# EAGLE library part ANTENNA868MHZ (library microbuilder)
868MHz Surface-Mount Antenna Digikey: ANT-868-SP_-ND
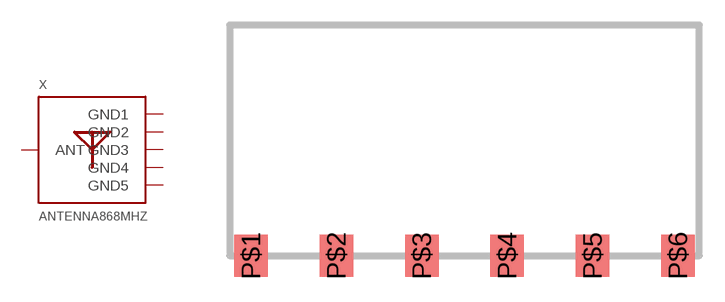
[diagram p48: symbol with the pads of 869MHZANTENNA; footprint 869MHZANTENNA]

Designator prefix X

## ANTENNA868MHZ  [869MHZANTENNA]
P$1  ANT
P$2  GND1  pwr
P$3  GND2  pwr
P$4  GND3  pwr
P$5  GND4  pwr
P$6  GND5  pwr

## Footprint 869MHZANTENNA (pad centres in mm)
smd 2 x 2.5: P$1 -12.7,-6.858; P$2 -7.62,-6.858; P$3 -2.54,-6.858; P$4 2.54,-6.858; P$5 7.62,-6.858; P$6 12.7,-6.858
